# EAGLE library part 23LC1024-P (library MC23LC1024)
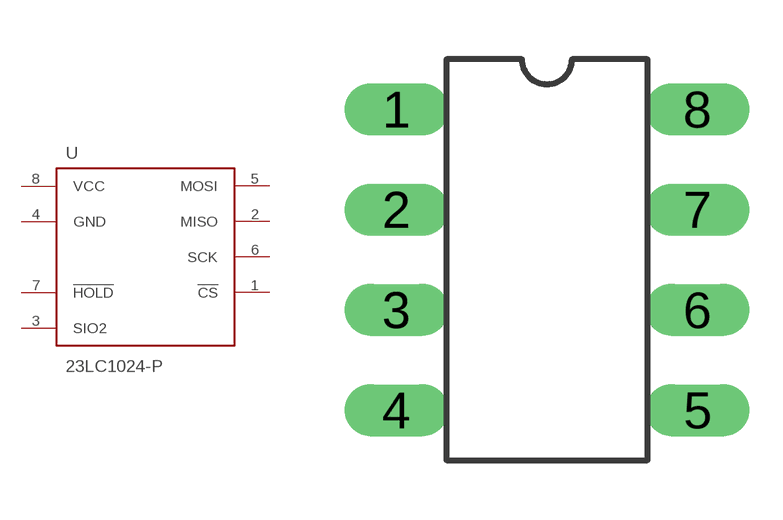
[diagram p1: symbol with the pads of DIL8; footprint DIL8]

Designator prefix -

## 23LC1024-P  [DIL8]
1  !CS!
2  MISO
3  SIO2
4  GND
5  MOSI
6  SCK
7  !HOLD!
8  VCC

## Footprint DIL8 (pad centres in mm)
Dual In Line package type P
drill 0.813 long: 1 -3.81,3.81; 2 -3.81,1.27; 3 -3.81,-1.27; 4 -3.81,-3.81; 5 3.81,-3.81; 6 3.81,-1.27; 7 3.81,1.27; 8 3.81,3.81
